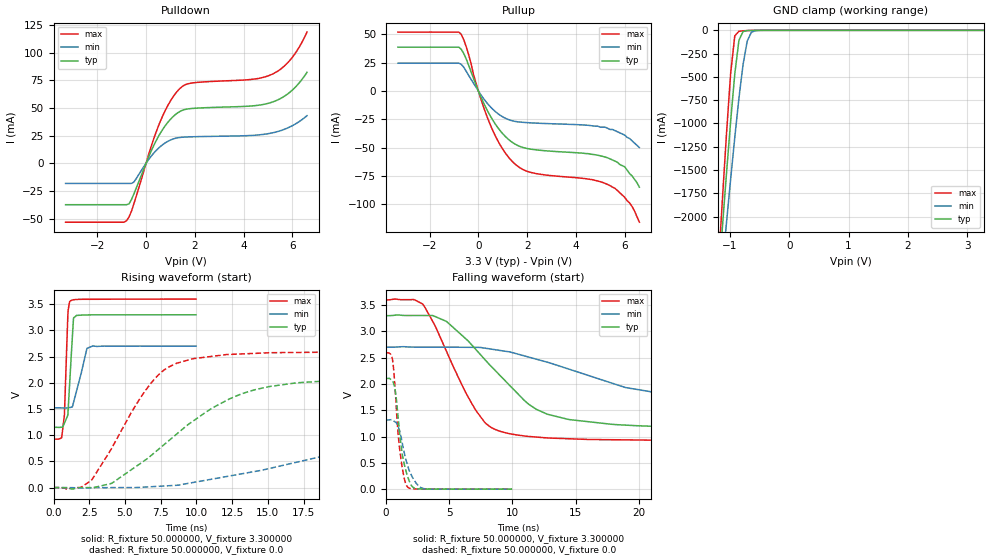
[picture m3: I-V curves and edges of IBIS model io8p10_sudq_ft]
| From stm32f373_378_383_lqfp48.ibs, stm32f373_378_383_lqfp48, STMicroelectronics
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|   Model io8p10_sudq_ft
[Model]  io8p10_sudq_ft
Model_type I/O
Polarity   Non-Inverting
Enable   Active-Low
Vinl =   0.990000V
Vinh =   2.310000V
Vmeas =  1.650000V
Cref =   50.000000pF
Rref =   100.000000M
Vref =   0.0V
C_comp   1.970900pF   1.892300pF   2.063200pF
[Temperature Range]   25.000000   0.125000k   -40.000000
[Pullup Reference]   3.300000V   2.700000V   3.600000V
[Pulldown Reference]   0.0V   0.0V   0.0V
[POWER Clamp Reference]   3.300000V   2.700000V   3.600000V
[GND Clamp Reference]   0.0V   0.0V   0.0V
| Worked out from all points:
|   slope of the pulldown table from 0 to 0.495 V, typ, clamps not added: 20.9 ohm
|   slope of the pullup table from 0 to 0.495 V, typ, clamps not added: 22.2 ohm
|   GND clamp passes 1 mA (typ) near -0.64 V on its own axis
|   rising waveform, R_fixture 50.000000, V_fixture 3.300000: 20-80 % time 274ps typ, 646ps min, 201ps max; typ from 1.15 V to 3.3 V
|   rising waveform, R_fixture 50.000000, V_fixture 0.0: 20-80 % time 6.37ns typ, 15.3ns min, 3.52ns max; typ from 0 V to 2.1 V
|   falling waveform, R_fixture 50.000000, V_fixture 3.300000: 20-80 % time 5.23ns typ, 11.3ns min, 3.26ns max; typ from 3.3 V to 1.15 V
|   falling waveform, R_fixture 50.000000, V_fixture 0.0: 20-80 % time 666ps typ, 883ps min, 542ps max; typ from 2.1 V to 0 V
[Pulldown]
|Voltage   I(typ)   I(min)   I(max)
-3.3V     -37.45mA   -18.2mA    -53.24mA
-800mV    -37.45mA   -18.2mA    -51.9mA
-700mV    -36.7mA    -18.2mA    -48.48mA
-500mV    -27.71mA   -17.01mA   -36.66mA
200mV     10.57mA    6.084mA    14.57mA
500mV     23.91mA    13.38mA    33.24mA
900mV     37.17mA    19.88mA    52.48mA
1.3V      45.55mA    23.01mA    65.5mA
1.8V      49.29mA    23.83mA    72.18mA
5.1V      54.68mA    27.07mA    79.72mA
5.9V      64.2mA     32.82mA    93.01mA
6.6V      82.13mA    42.97mA    118.4mA
[Pullup]
|Voltage   I(typ)   I(min)   I(max)
-3.3V     38.74mA    24.61mA    52.11mA
-800mV    38.74mA    24.61mA    52.11mA
-500mV    28.37mA    17.48mA    39.19mA
0V        90fA       16pA       0A
500mV     -22.5mA    -14.16mA   -30.52mA
900mV     -35.28mA   -21.55mA   -48mA
1.4V      -45.55mA   -26.41mA   -62.54mA
2.2V      -51.57mA   -28.22mA   -72.25mA
5.4V      -60mA      -34mA      -83.7mA
6V        -67mA      -39mA      -94mA
6.2V      -73mA      -42mA      -99mA
6.6V      -85mA      -50mA      -116mA
[GND_clamp]
|Voltage   I(typ)   I(min)   I(max)
-3.3V     -9.525A    -9.501A    -9.513A
-1.2V     -2.719A    -3.023A    -2.568A
-1.13V    -2.122A    -2.541A    -1.826A
-1.06V    -1.537A    -2.065A    -1.111A
-990mV    -975.7mA   -1.599A    -462mA
-920mV    -467.4mA   -1.149A    -59mA
-850mV    -106.6mA   -727.3mA   -10.11mA
-780mV    -13.06mA   -365.4mA   -5.254mA
-710mV    -3.045mA   -114.8mA   -2.635mA
-640mV    -943.2uA   -20.16mA   -905.7uA
-570mV    -199.4uA   -3.959mA   -156.8uA
3.28V     0A         0A         0A
[POWER_clamp]
|Voltage   I(typ)   I(min)   I(max)
-3.28V    0A         0A         0A
0V        0A         0A         0A
[Ramp]
| variable   typ   min   max
dV/dt_r  1.26234/6.36252n   0.77934/15.28583n   1.55466/3.52049n
dV/dt_f  1.28940/5.22957n   0.69930/11.29258n   1.60466/3.25246n
R_load = 50.000000
[Rising Waveform]
R_fixture= 50.000000
V_fixture= 3.300000
V_fixture_min= 2.700000
V_fixture_max= 3.600000
|time   V(typ)   V(min)   V(max)
0s        1.151V     1.522V     925.5mV
560.6ps   1.153V     1.522V     948.1mV
760.8ps   1.229V     1.52V      1.381V
1.001ns   1.383V     1.523V     3.288V
1.141ns   2.05V      1.53V      3.556V
1.401ns   3.24V      1.627V     3.587V
1.622ns   3.289V     1.857V     3.592V
2.342ns   3.297V     2.659V     3.596V
2.743ns   3.298V     2.704V     3.596V
9.97ns    3.3V       2.7V       3.6V
[Rising Waveform]
R_fixture= 50.000000
V_fixture= 0.0
V_fixture_min= 0.0
V_fixture_max= 0.0
|time   V(typ)   V(min)   V(max)
0s        -32.88uV   -23.39uV   -20.28uV
2.603ns   -251.3uV   -5.333mV   130.3mV
4.104ns   87.73mV    -418.2uV   769.3mV
7.007ns   653.9mV    19.5mV     2.055V
8.008ns   883.3mV    34.83mV    2.295V
9.81ns    1.279V     99.64mV    2.463V
13.01ns   1.774V     255.7mV    2.551V
17.02ns   2.001V     485.3mV    2.58V
32.23ns   2.101V     1.164V     2.591V
49.85ns   2.104V     1.316V     2.591V
[Falling Waveform]
R_fixture= 50.000000
V_fixture= 3.300000
V_fixture_min= 2.700000
V_fixture_max= 3.600000
|time   V(typ)   V(min)   V(max)
0s        3.3V       2.7V       3.6V
2.903ns   3.303V     2.701V     3.521V
4.805ns   3.187V     2.701V     2.614V
7.107ns   2.657V     2.697V     1.5V
8.208ns   2.363V     2.668V     1.192V
9.61ns    2.017V     2.617V     1.064V
12.71ns   1.431V     2.418V     974.9mV
17.82ns   1.234V     2.02V      940.3mV
24.72ns   1.174V     1.703V     927.7mV
49.85ns   1.151V     1.522V     925.5mV
[Falling Waveform]
R_fixture= 50.000000
V_fixture= 0.0
V_fixture_min= 0.0
V_fixture_max= 0.0
|time   V(typ)   V(min)   V(max)
0s        2.104V     1.316V     2.591V
520.5ps   2.062V     1.315V     2.469V
760.8ps   1.844V     1.273V     1.805V
961ps     1.385V     1.194V     1.072V
1.081ns   1.075V     1.115V     780.6mV
1.461ns   465.1mV    685.3mV    196.5mV
1.722ns   240.9mV    449.7mV    37.83mV
2.162ns   31.83mV    202.6mV    6.415mV
3.003ns   2.6mV      9.671mV    2.044mV
9.97ns    -32.88uV   -23.39uV   -20.28uV
